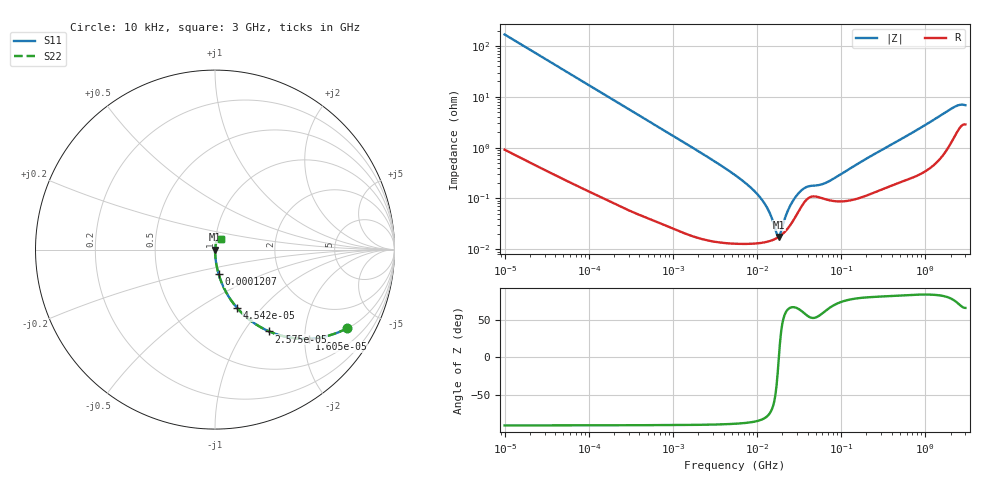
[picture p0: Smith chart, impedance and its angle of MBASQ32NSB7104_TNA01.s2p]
! MBASQ32NSB7104_TNA01  S-PARAMETER MODEL  ( Standard Model )
! Model Generated by TAIYO YUDEN Corporation (http://www.ty-top.com)
! Version 1.0
! TAIYO YUDEN Control No. 220601
! Copyright(c) 2013 TAIYO YUDEN CO.,LTD. All Rights Reserved.
! Product Description (link to TY-COMPAS)
! https://ds.yuden.co.jp/TYCOMPAS/or/detail?pn=MBASQ32NSB7104KTNA01&u=M
! Products Name : Multilayer Ceramic Capacitors
! Characteristics :
!  Capacitance : 0.1 [uF] , Rated Voltage : 250 [V] , TCC : X7R
!  Case Size : 3.2 x 2.5 / 0.126 x 0.098 [mm/inch] , Thickness : 1.9 / 0.075 [mm/inch]
!  (Conditions: Temperature = 25 [degC] , DC Bias Voltage = 0 [V])
! External Node Assignments :
!  1  o---| |---o  2
! GND o---------o GND
! Frequency Range : 10kHz  -  3GHz  [ 401 STEP ]
# MHZ S RI R 50
! Freq[MHz].  S11 Real  S11 Imag  S21 Real  S21 Imag  S12 Real  S12 Imag  S22 Real  S22 Imag
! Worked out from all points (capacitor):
!   401 points, 10 kHz to 3 GHz, reference 50 ohm
!   read as one part in series: C = 94.5 nF near 10.65 kHz
!   lowest |Z| = 17.5 mohm at 18.15 MHz (marker M1)
!   series resonance near 18.18 MHz, so ESL is about 810 pH
!   S11 on the Smith chart (normalised r, x): 10 kHz: 1.02, -3.36; 16.05 kHz: 1.01, -2.10; 25.75 kHz: 1.01, -1.31; 45.42 kHz: 1.01, -0.74; 120.7 kHz: 1.00, -0.28; 3 GHz: 1.06, +0.12
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0.01  0.7377 -0.4372  0.2623 0.4372  0.2623 0.4372  0.7377 -0.4372
0.016047  0.5241 -0.4965  0.4759 0.4965  0.4759 0.4965  0.5241 -0.4965
0.02575  0.3016 -0.4558  0.6984 0.4558  0.6984 0.4558  0.3016 -0.4558
0.045421  0.1235 -0.3255  0.8765 0.3255  0.8765 0.3255  0.1235 -0.3255
0.082683  0.0418 -0.1962  0.9582 0.1962  0.9582 0.1962  0.0418 -0.1962
0.120707  0.0205 -0.1377  0.9795 0.1377  0.9795 0.1377  0.0205 -0.1377
0.683653  0.000959 -0.025  0.999 0.025  0.999 0.025  0.000959 -0.025
5.477226  0.000137 -0.00289  0.9999 0.00289  0.9999 0.00289  0.000137 -0.00289
8.516475  0.000131 -0.00161  0.9999 0.00161  0.9999 0.00161  0.000131 -0.00161
11.31085  0.000135 -0.00096  0.9999 0.00096  0.9999 0.00096  0.000135 -0.00096
13.66633  0.000143 -0.000569  0.9999 0.000569  0.9999 0.000569  0.000143 -0.000569
17.04125  0.000165 -0.000129  0.9998 0.000129  0.9998 0.000129  0.000165 -0.000129
18.15044  0.000175 -2.96e-06  0.9998 2.96e-06  0.9998 2.96e-06  0.000175 -2.96e-06
19.33182  0.000189 0.000125  0.9998 -0.000125  0.9998 -0.000125  0.000189 0.000125
23.35767  0.00026 0.000523  0.9997 -0.000523  0.9997 -0.000523  0.00026 0.000523
28.22191  0.000418 0.000937  0.9996 -0.000937  0.9996 -0.000937  0.000418 0.000937
35.19136  0.000773 0.00132  0.9992 -0.00132  0.9992 -0.00132  0.000773 0.00132
45.28751  0.00109 0.0014  0.9989 -0.0014  0.9989 -0.0014  0.00109 0.0014
70.41703  0.000934 0.00193  0.9991 -0.00193  0.9991 -0.00193  0.000934 0.00193
374.4521  0.00183 0.0107  0.9982 -0.0107  0.9982 -0.0107  0.00183 0.0107
2120.803  0.0173 0.057  0.9827 -0.057  0.9827 -0.057  0.0173 0.057
3000  0.0313 0.0585  0.9687 -0.0585  0.9687 -0.0585  0.0313 0.0585
